FUNCTION_BLOCK FB31
TITLE =Find Home
//*****************************************************************************
//* maxon motor ag
//* R&D
//* all rights reserved
//*****************************************************************************
//* Summary:  Find Home
//*
//* Remarks:
//*
//* Created under: STEP7 REV5.2+SP1
//*****************************************************************************
//* History:
//* 19.05.2004 | INA   first release
//*
//*
//*****************************************************************************
//

AUTHOR:INA
FAMILY:HomingMo
NAME:FindHome
VERSION:00.01


VAR_INPUT

Write : BOOL //A rising edge start the command

  NodeID : BYTE //Adress of the maxon device

  HomingMethod : INT //Homing Method

END_VAR
VAR_OUTPUT
  Done : BOOL //Data valid flag is TRUE if data were available

  Err : BOOL //Error flag is TRUE if an Error has occured, see ErrNo for more details

  ErrNo : DINT //Contains detailed error information

END_VAR
VAR
  xEdgeMerker : BOOL //Edge Merker

  xEdgeFlag : BOOL //Edge Flag

  xStep : INT
  xEnableOperation : WORD  := W#16#F
  xAbsolutePosition : WORD  := W#16#1F
END_VAR

BEGIN

NETWORK
TITLE = Activate the service function
//

// SDO Write "Find Home"

       U    #Write
       FP   #xEdgeFlag                   // recognize a positiv edge of the Read signal
       =    #xEdgeMerker                 // and set the xEdgeMerker for one cycle to true

       L    #xStep
       L    0
       ==I
       U    #xEdgeMerker
       SPB  nstp                         // iStep = 1 -> fnc1

       L    #xStep                       // jump list
       SPL  List
       SPA  rdef
       SPA  fnc1
       SPA  fncE
List  :SPA  rdef

rdef  :NOP  0
       R    #Done                        // reset Done
       R    #Err
       L    0
       T    #xStep                       // iStep = 0
       SPA  end

fnc1  :NOP  0
       CALL FC12
         NodeID:=#NodeID
         Index:=DW#16#000060F6
         SubIndex:=DW#16#00000001
         ValueIn:=#HomingMethod
         RET_VAL:=#Done
         Err:=#Err
         ErrNo:=#ErrNo

       L    1
       U    #Err
       SPB  fncE

       NOP  0
       CALL FC15
         NodeID:=#NodeID
         Index:=DW#16#00006040
         SubIndex:=DW#16#00000000
         ValueIn:=#xEnableOperation
         RET_VAL:=#Done
         Err:=#Err
         ErrNo:=#ErrNo

       L    1
       U    #Err
       SPB  fncE

       NOP  0
       CALL FC15
         NodeID:=#NodeID
         Index:=DW#16#00006040
         SubIndex:=DW#16#00000000
         ValueIn:=#xAbsolutePosition
         RET_VAL:=#Done
         Err:=#Err
         ErrNo:=#ErrNo

fncE  :NOP  0
       L    0
       T    #xStep
       SPA  end

nstp  :NOP  0
       L    #xStep
       INC            1
       T    #xStep

end   :NOP  0
END_FUNCTION_BLOCK
